DATA_BLOCK DB112
TITLE =

AUTHOR:INA
FAMILY:Velocity
NAME:nb
VERSION:00.00


    FB112


BEGIN
       Write:=FALSE
       NodeID:=B#16#00
       VelocityMust:=L#0
       Done:=FALSE
       Err:=FALSE
       ErrNo:=L#0
       xEdgeMerker:=FALSE
       xEdgeFlag:=FALSE
       xStep:=0

END_DATA_BLOCK
